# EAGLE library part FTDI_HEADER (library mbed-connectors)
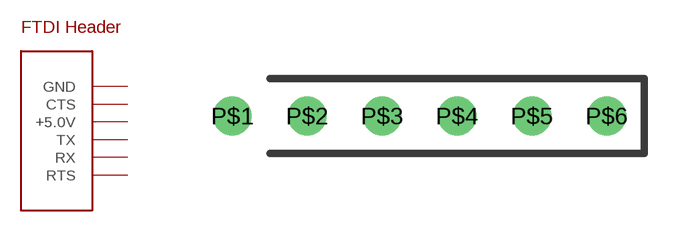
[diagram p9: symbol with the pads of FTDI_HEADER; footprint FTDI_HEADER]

Designator prefix CON

## FTDI_HEADER  [FTDI_HEADER]
P$1  GND
P$2  CTS
P$3  +5.0V
P$4  TX
P$5  RX
P$6  RTS

## Footprint FTDI_HEADER (pad centres in mm)
drill 0.8: P$1 0,0; P$2 2.54,0; P$3 5.08,0; P$4 7.62,0; P$5 10.16,0; P$6 12.7,0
